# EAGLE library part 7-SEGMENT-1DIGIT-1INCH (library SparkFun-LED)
7-Segment Display, single digit, 1" EZ is for kits. Pads are only exposed on the bottom side to help prevent soldering in upside down. Datasheet (Red) Datasheet (Blue) SparkFun Products 7-Segment Display - LED (Red) (COM-08546) 7-Segment Display - LED (Blue) (COM-09191)
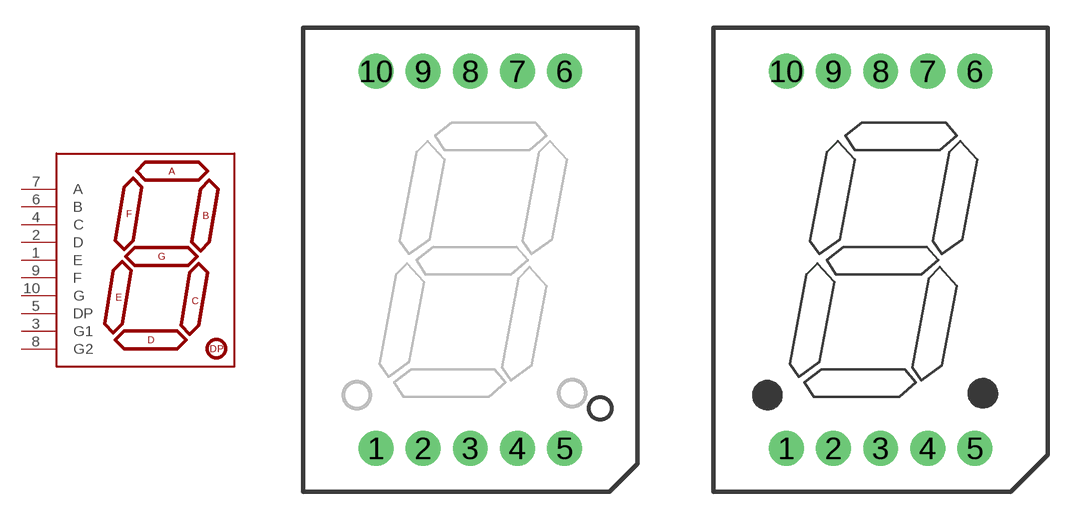
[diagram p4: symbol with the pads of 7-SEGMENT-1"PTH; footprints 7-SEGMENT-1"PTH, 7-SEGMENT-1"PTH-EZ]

Designator prefix -

## 7-SEGMENT-1DIGIT-1INCH-RED (PROD_ID: COMP-08615; VALUE: YSD-1601AR4B-8)  [7-SEGMENT-1"PTH]
1  E
2  D
3  G1
4  C
5  DP
6  B
7  A
8  G2
9  F
10  G

## 7-SEGMENT-1DIGIT-1INCH-RED-EZ (PROD_ID: COMP-08615; VALUE: YSD-1601AR4B-8)  [7-SEGMENT-1"PTH-EZ]
Pads as for 7-SEGMENT-1"PTH

## 7-SEGMENT-1DIGIT-1INCH-BLUE (PROD_ID: COMP-09495; VALUE: YSD-160AB3C-8)  [7-SEGMENT-1"PTH]
Pads as for 7-SEGMENT-1"PTH

## 7-SEGMENT-1DIGIT-1INCH-BLUE-EZ (PROD_ID: COMP-09495; VALUE: YSD-160AB3C-8)  [7-SEGMENT-1"PTH-EZ]
Pads as for 7-SEGMENT-1"PTH

## Footprint 7-SEGMENT-1"PTH (pad centres in mm)
7 Segment display Storefront SKU#: COM-08546
drill 1 pad 1.88: 1 -5.08,-10.16; 2 -2.54,-10.16; 3 0,-10.16; 4 2.54,-10.16; 5 5.08,-10.16; 6 5.08,10.16; 7 2.54,10.16; 8 0,10.16; 9 -2.54,10.16; 10 -5.08,10.16

## Footprint 7-SEGMENT-1"PTH-EZ (pad centres in mm)
drill 1 pad 1.88: 1 -5.08,-10.16; 2 -2.54,-10.16; 3 0,-10.16; 4 2.54,-10.16; 5 5.08,-10.16; 6 5.08,10.16; 7 2.54,10.16; 8 0,10.16; 9 -2.54,10.16; 10 -5.08,10.16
